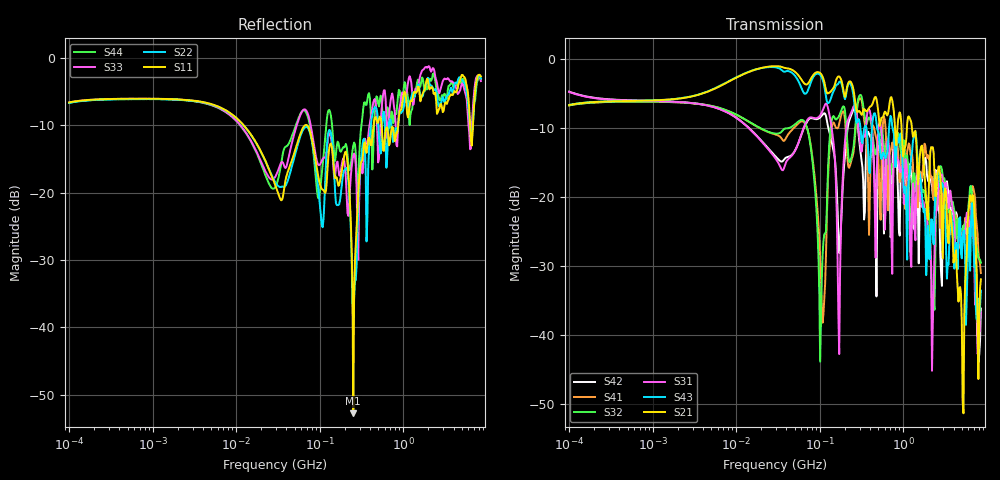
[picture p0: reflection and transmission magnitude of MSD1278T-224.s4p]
# MHz S MA R 50
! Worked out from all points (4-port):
!   498 points, 100 kHz to 8.5 GHz, reference 50 ohm
!   strongest paths, dB at 100 kHz, 1.698 MHz, 29.49 MHz, 500.7 MHz, 8.5 GHz:
!     S21: -6.7, -5.9, -1.1, -7.5, -31.9
!     S43: -6.7, -5.9, -1.2, -10.5, -33.6
!     S31: -4.8, -6.2, -14.4, -10.6, -36.8
!     S32: -6.8, -6.3, -10.8, -12.4, -29.5
!     S41: -6.8, -6.3, -11.0, -14.0, -31.0
!     S42: -4.8, -6.2, -14.1, -14.2, -36.2
!   lowest |S11| = -52.7 dB at 252.3 MHz (marker M1), VSWR 1.00, Z = 50.2 - j0.167 ohm
!   |S11| at or under -10 dB: 70.57 MHz to 441.6 MHz (371 MHz wide, 145 % of centre); 550.9 MHz to 869.6 MHz (318.7 MHz wide, 44.9 % of centre); 6.319 GHz to 6.829 GHz (509.7 MHz wide, 7.75 % of centre)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
0.1  0.4674 18.9  0.4625 20.2  0.5757 -16.2  0.4596 -160.9
     0.4625 20.2  0.4637 19.1  0.4595 -160.8  0.5782 -16.2
     0.5757 -16.2  0.4595 -160.8  0.4664 19.0  0.4633 20.1
     0.4596 -160.9  0.5782 -16.2  0.4633 20.1  0.4634 19.2
64.10508  0.308 -8.9  0.671 -22.0  0.3159 155.7  0.3491 7.4
          0.671 -22.0  0.2969 -10.8  0.3563 7.4  0.3116 153.1
          0.3159 155.7  0.3563 7.4  0.4128 -5.8  0.5696 -26.4
          0.3491 7.4  0.3116 153.1  0.5696 -26.4  0.4098 -8.5
101.2184  0.1138 -43.5  0.7884 -30.5  0.3894 56.6  0.03644 -92.1
          0.7884 -30.5  0.07582 -53.2  0.006412 -131.2  0.3761 46.9
          0.3894 56.6  0.006412 -131.2  0.1622 -20.7  0.7633 -36.9
          0.03644 -92.1  0.3761 46.9  0.7633 -36.9  0.1045 14.7
171.1518  0.1142 -32.0  0.7443 -39.0  0.007274 51.6  0.3387 39.4
          0.7443 -39.0  0.08211 -31.1  0.3874 31.3  0.0392 -171.6
          0.007274 51.6  0.3874 31.3  0.1341 -26.7  0.6798 -43.6
          0.3387 39.4  0.0392 -171.6  0.6798 -43.6  0.2165 -17.8
252.3442  0.002304 -46.2  0.6062 -67.4  0.4471 2.3  0.2063 20.6
          0.6062 -67.4  0.0109 99.2  0.2244 19.3  0.4273 2.5
          0.4471 2.3  0.2244 19.3  0.188 -2.0  0.5509 -87.6
          0.2063 20.6  0.4273 2.5  0.5509 -87.6  0.224 1.3
2016.336  0.617 -173.3  0.1045 165.4  0.04075 117.9  0.1895 139.9
          0.1045 165.4  0.7034 -170.2  0.08008 104.8  0.1286 149.6
          0.04075 117.9  0.08008 104.8  0.8682 -172.8  0.04689 144.3
          0.1895 139.9  0.1286 149.6  0.04689 144.3  0.66 -164.1
8500  0.7295 -54.7  0.02527 -44.2  0.01453 -33.0  0.02807 -139.1
      0.02527 -44.2  0.704 -56.4  0.03336 -133.2  0.01554 -51.9
      0.01453 -33.0  0.03336 -133.2  0.6729 -53.2  0.02095 -28.8
      0.02807 -139.1  0.01554 -51.9  0.02095 -28.8  0.6952 -52.7
